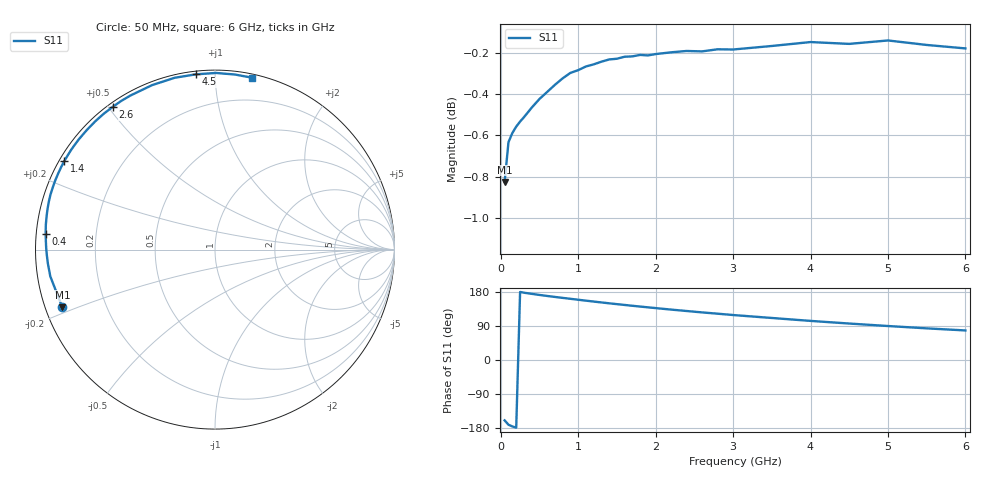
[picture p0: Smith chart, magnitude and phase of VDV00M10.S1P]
! Infineon Technologies  Discrete & RF Semiconductors
! BBY 55-03
! Si Tuning Diode in SOD323
! VR =
! S-Parameters:  June  1999
# GHz  S  MA  R  50
!  f  S11
! GHz  MAG  ANG
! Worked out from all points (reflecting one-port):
!   34 points, 50 MHz to 6 GHz, reference 50 ohm
!   lowest |S11| = -0.8 dB at 50 MHz (marker M1), VSWR 21.03, Z = 2.46 - j9.11 ohm
!   phase of S11 starts at -159 deg and turns -123 deg over the sweep
!   S11 on the Smith chart (normalised r, x): 50 MHz: 0.05, -0.18; 400 MHz: 0.03, +0.05; 1.4 GHz: 0.01, +0.27; 2.6 GHz: 0.01, +0.51; 4.5 GHz: 0.02, +0.90; 6 GHz: 0.03, +1.23
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0.05  0.9092 -159.3
0.1  0.9298 -170.8
0.15  0.9345 -175.4
0.2  0.9379 -178.4
0.25  0.9405 179.5
0.3  0.9428 177.6
0.4  0.9479 174.6
0.5  0.9525 171.7
0.6  0.9563 169.0
0.8  0.9636 163.9
0.9  0.9665 161.5
1.1  0.97 156.6
1.2  0.9711 154.2
1.4  0.9738 149.6
1.6  0.9753 145.3
1.8  0.9763 141.0
2  0.9767 137.0
2.2  0.9777 133.0
2.4  0.9784 129.3
2.6  0.9782 125.6
2.8  0.9793 122.2
3  0.9792 118.7
3.5  0.9811 110.9
4  0.9833 103.2
4.5  0.9823 96.2
5  0.9842 89.7
5.5  0.9817 83.5
6  0.9798 78.0
